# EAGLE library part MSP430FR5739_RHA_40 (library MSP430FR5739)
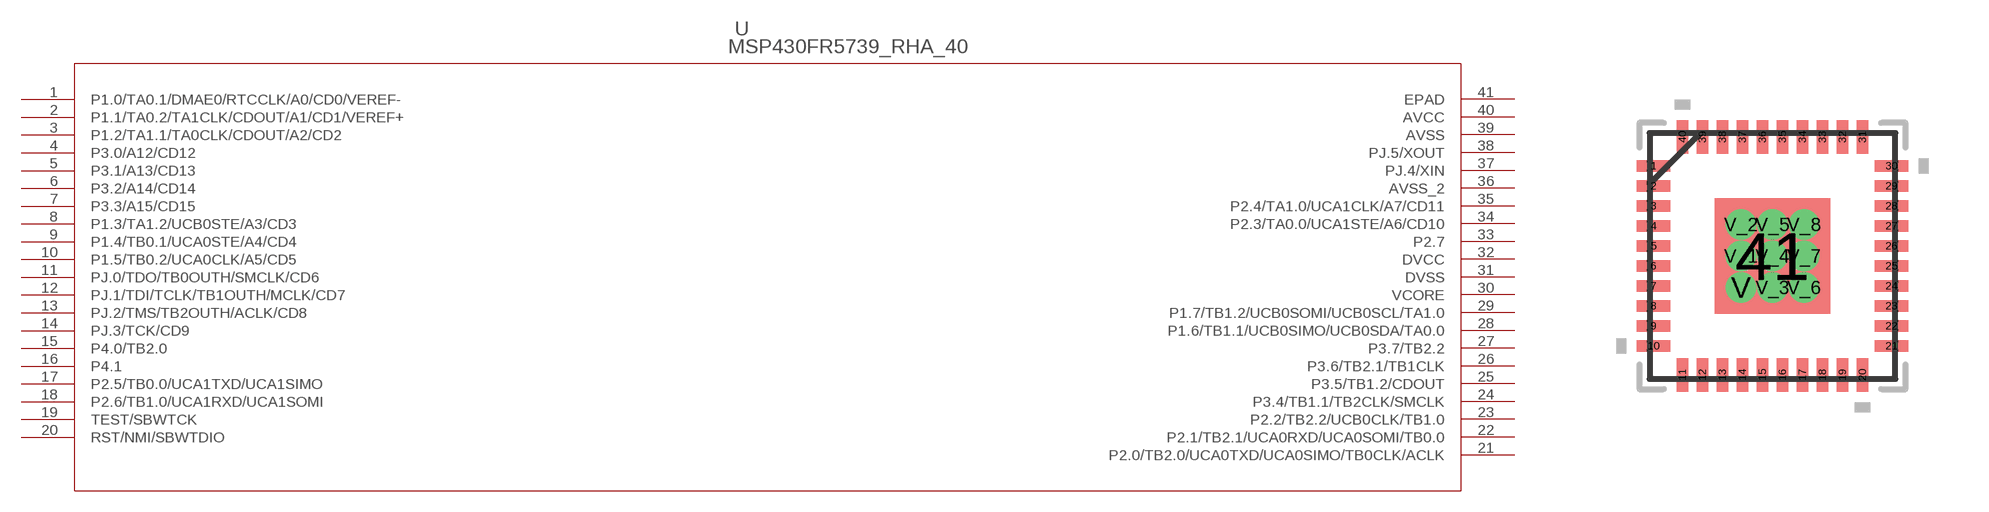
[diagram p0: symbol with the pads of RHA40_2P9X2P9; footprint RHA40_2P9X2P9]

Designator prefix U

## MSP430FR5739_RHA_40 (DATASHEETURL: http://www.ti.com/lit/gpn/MSP430FR5739; DESCRIPTION: MSP430FR573x,MSP430FR572x Mixed Signal Microcontroller; FAMILY_NAME: FRAM Series; GENERIC_PART_NUMBER: MSP430FR5739; INDUSTRY_STD_PKG_TYPE: VQFN; MANUFACTURER: Texas Instruments; MANUFACTURER_PART_NUMBER: msp430fr5739_rha_40; PACKAGE_DESIGNATOR: RHA; PIN_COUNT: 40; VENDOR: Texas Instruments)  [RHA40_2P9X2P9]
1  P1.0/TA0.1/DMAE0/RTCCLK/A0/CD0/VEREF-
2  P1.1/TA0.2/TA1CLK/CDOUT/A1/CD1/VEREF+
3  P1.2/TA1.1/TA0CLK/CDOUT/A2/CD2
4  P3.0/A12/CD12
5  P3.1/A13/CD13
6  P3.2/A14/CD14
7  P3.3/A15/CD15
8  P1.3/TA1.2/UCB0STE/A3/CD3
9  P1.4/TB0.1/UCA0STE/A4/CD4
10  P1.5/TB0.2/UCA0CLK/A5/CD5
11  PJ.0/TDO/TB0OUTH/SMCLK/CD6
12  PJ.1/TDI/TCLK/TB1OUTH/MCLK/CD7
13  PJ.2/TMS/TB2OUTH/ACLK/CD8
14  PJ.3/TCK/CD9
15  P4.0/TB2.0
16  P4.1
17  P2.5/TB0.0/UCA1TXD/UCA1SIMO
18  P2.6/TB1.0/UCA1RXD/UCA1SOMI
19  TEST/SBWTCK
20  RST/NMI/SBWTDIO
21  P2.0/TB2.0/UCA0TXD/UCA0SIMO/TB0CLK/ACLK
22  P2.1/TB2.1/UCA0RXD/UCA0SOMI/TB0.0
23  P2.2/TB2.2/UCB0CLK/TB1.0
24  P3.4/TB1.1/TB2CLK/SMCLK
25  P3.5/TB1.2/CDOUT
26  P3.6/TB2.1/TB1CLK
27  P3.7/TB2.2
28  P1.6/TB1.1/UCB0SIMO/UCB0SDA/TA0.0
29  P1.7/TB1.2/UCB0SOMI/UCB0SCL/TA1.0
30  VCORE  pwr
31  DVSS  pwr
32  DVCC  pwr
33  P2.7
34  P2.3/TA0.0/UCA1STE/A6/CD10
35  P2.4/TA1.0/UCA1CLK/A7/CD11
36  AVSS_2  pwr
37  PJ.4/XIN
38  PJ.5/XOUT
39  AVSS  pwr
40  AVCC  pwr
41  EPAD  pas

## Footprint RHA40_2P9X2P9 (pad centres in mm)
smd 0.838 x 0.279: 1 -2.975,2.25; 2 -2.975,1.75; 3 -2.975,1.25; 4 -2.975,0.75; 5 -2.975,0.25; 6 -2.975,-0.25; 7 -2.975,-0.75; 8 -2.975,-1.25; 9 -2.975,-1.75; 10 -2.975,-2.25; 21 2.975,-2.25; 22 2.975,-1.75; 23 2.975,-1.25; 24 2.975,-0.75; 25 2.975,-0.25; 26 2.975,0.25; 27 2.975,0.75; 28 2.975,1.25; 29 2.975,1.75; 30 2.975,2.25
smd 0.279 x 0.838: 11 -2.251,-2.975; 12 -1.75,-2.975; 13 -1.25,-2.975; 14 -0.75,-2.975; 15 -0.25,-2.975; 16 0.25,-2.975; 17 0.75,-2.975; 18 1.25,-2.975; 19 1.75,-2.975; 20 2.251,-2.975; 31 2.251,2.975; 32 1.75,2.975; 33 1.25,2.975; 34 0.75,2.975; 35 0.25,2.975; 36 -0.25,2.975; 37 -0.75,2.975; 38 -1.25,2.975; 39 -1.75,2.975; 40 -2.251,2.975
smd 2.896 x 2.896: 41 0,0
drill 0.254: V -0.787,-0.787; V_1 -0.787,0; V_2 -0.787,0.787; V_3 0,-0.787; V_4 0,0; V_5 0,0.787; V_6 0.787,-0.787; V_7 0.787,0; V_8 0.787,0.787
